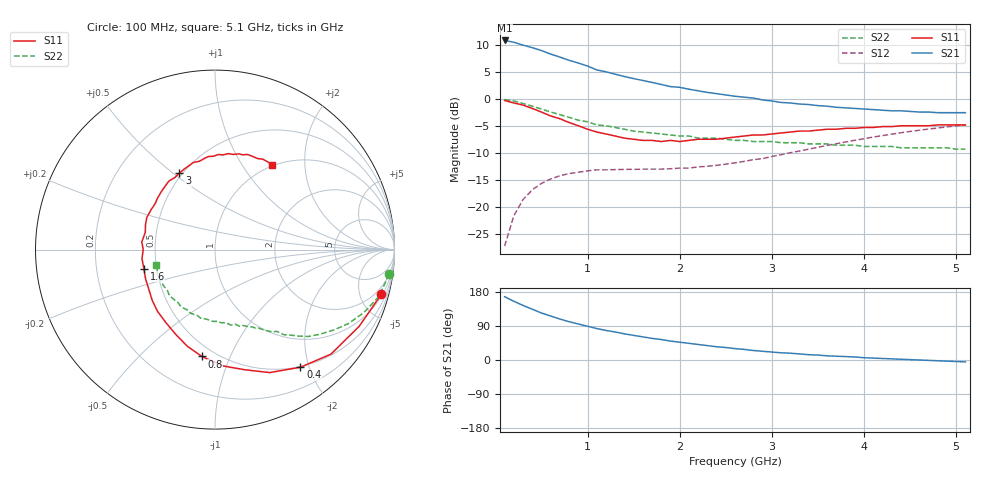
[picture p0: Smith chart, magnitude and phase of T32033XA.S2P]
!AT-32033
!S PARAMETERS at Vce=0.3 V  Ic=1mA.  LAST UPDATED 01-05-95
# ghz s ma r 50
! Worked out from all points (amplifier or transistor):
!   51 points, 100 MHz to 5.1 GHz, reference 50 ohm
!   highest |S21| = 10.8 dB at 100 MHz (marker M1)
!   |S21| within 3 dB of that: start of sweep to 685.6 MHz
!   unconditionally stable (mu >= 1): 1.627 GHz to end of sweep
!   at 900 MHz: K = 0.60, MSG = 10.1 dB, |S12| = -13.6 dB
!   at 2.6 GHz: K = 1.22, MAG = 3.4 dB, |S12| = -11.9 dB
!   at 5.1 GHz: K = 1.02, MAG = 0.3 dB, |S12| = -4.9 dB
!   S11 on the Smith chart (normalised r, x): 100 MHz: 1.17, -7.41; 400 MHz: 0.49, -1.86; 800 MHz: 0.42, -0.79; 1.6 GHz: 0.42, -0.11; 3 GHz: 0.48, +0.53; 5.1 GHz: 0.98, +1.37
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0.1  0.96 -15.0  3.45 167.0  0.043 82.0  0.98 -8.0
0.2  0.91 -28.0  3.32 155.0  0.082 71.0  0.95 -16.0
0.3  0.87 -42.0  3.12 144.0  0.116 63.0  0.9 -23.0
0.4  0.81 -54.0  2.96 134.0  0.143 56.0  0.85 -29.0
0.5  0.75 -66.0  2.78 124.0  0.164 50.0  0.8 -34.0
0.6  0.69 -76.0  2.58 116.0  0.18 45.0  0.75 -39.0
0.7  0.65 -86.0  2.42 108.0  0.193 41.0  0.71 -43.0
0.8  0.6 -97.0  2.26 101.0  0.202 37.0  0.67 -46.0
1  0.52 -115.0  2 89.0  0.214 32.0  0.61 -51.0
1.1  0.49 -124.0  1.84 83.0  0.219 29.0  0.57 -53.0
1.2  0.47 -133.0  1.77 78.0  0.219 28.0  0.56 -55.0
1.4  0.43 -149.0  1.6 69.0  0.221 27.0  0.52 -59.0
1.6  0.41 -165.0  1.47 61.0  0.222 26.0  0.49 -63.0
1.8  0.4 -180.0  1.35 54.0  0.222 26.0  0.47 -66.0
1.9  0.41 174.0  1.29 50.0  0.224 26.0  0.46 -68.0
2  0.4 166.0  1.27 47.0  0.227 28.0  0.45 -70.0
2.3  0.42 148.0  1.14 38.0  0.236 30.0  0.43 -76.0
2.6  0.44 133.0  1.05 30.0  0.254 33.0  0.41 -83.0
3  0.47 115.0  0.95 21.0  0.291 36.0  0.4 -92.0
3.5  0.51 97.0  0.86 13.0  0.354 35.0  0.38 -108.0
4.3  0.55 74.0  0.77 3.0  0.468 28.0  0.36 -135.0
5.1  0.57 56.0  0.74 -5.0  0.57 17.0  0.34 -165.0
